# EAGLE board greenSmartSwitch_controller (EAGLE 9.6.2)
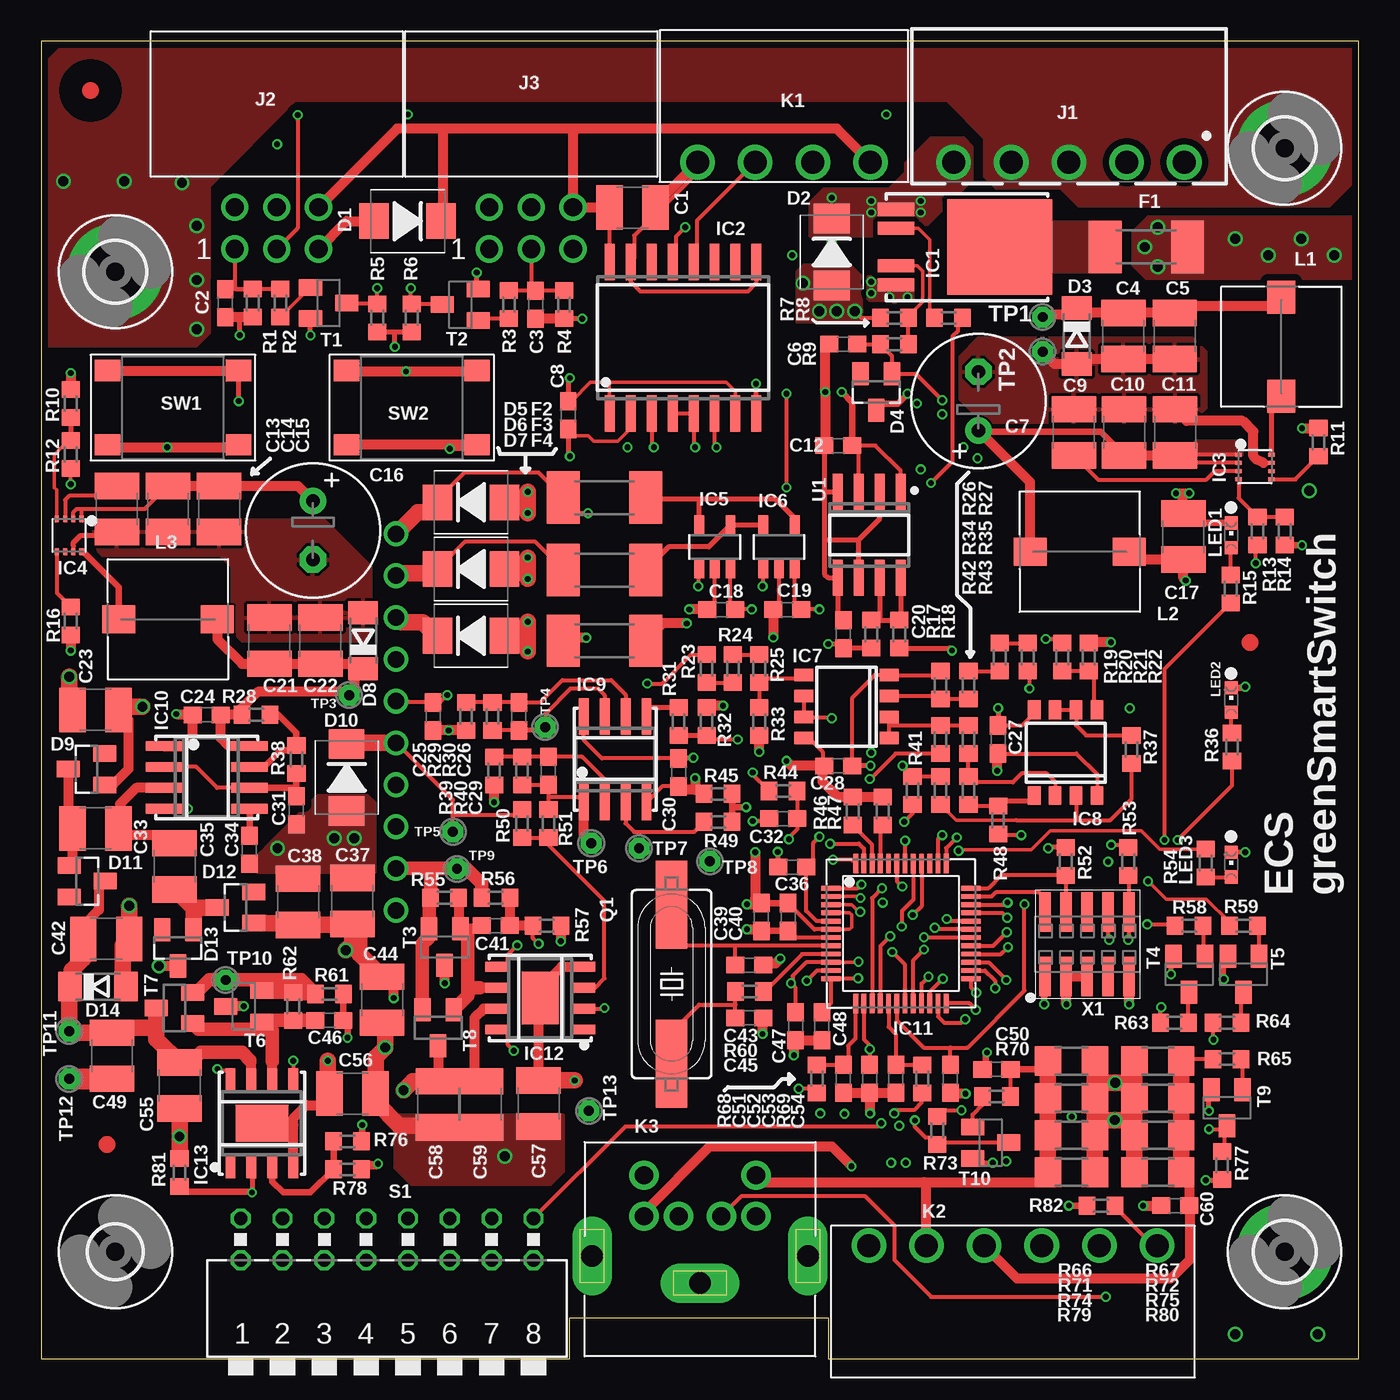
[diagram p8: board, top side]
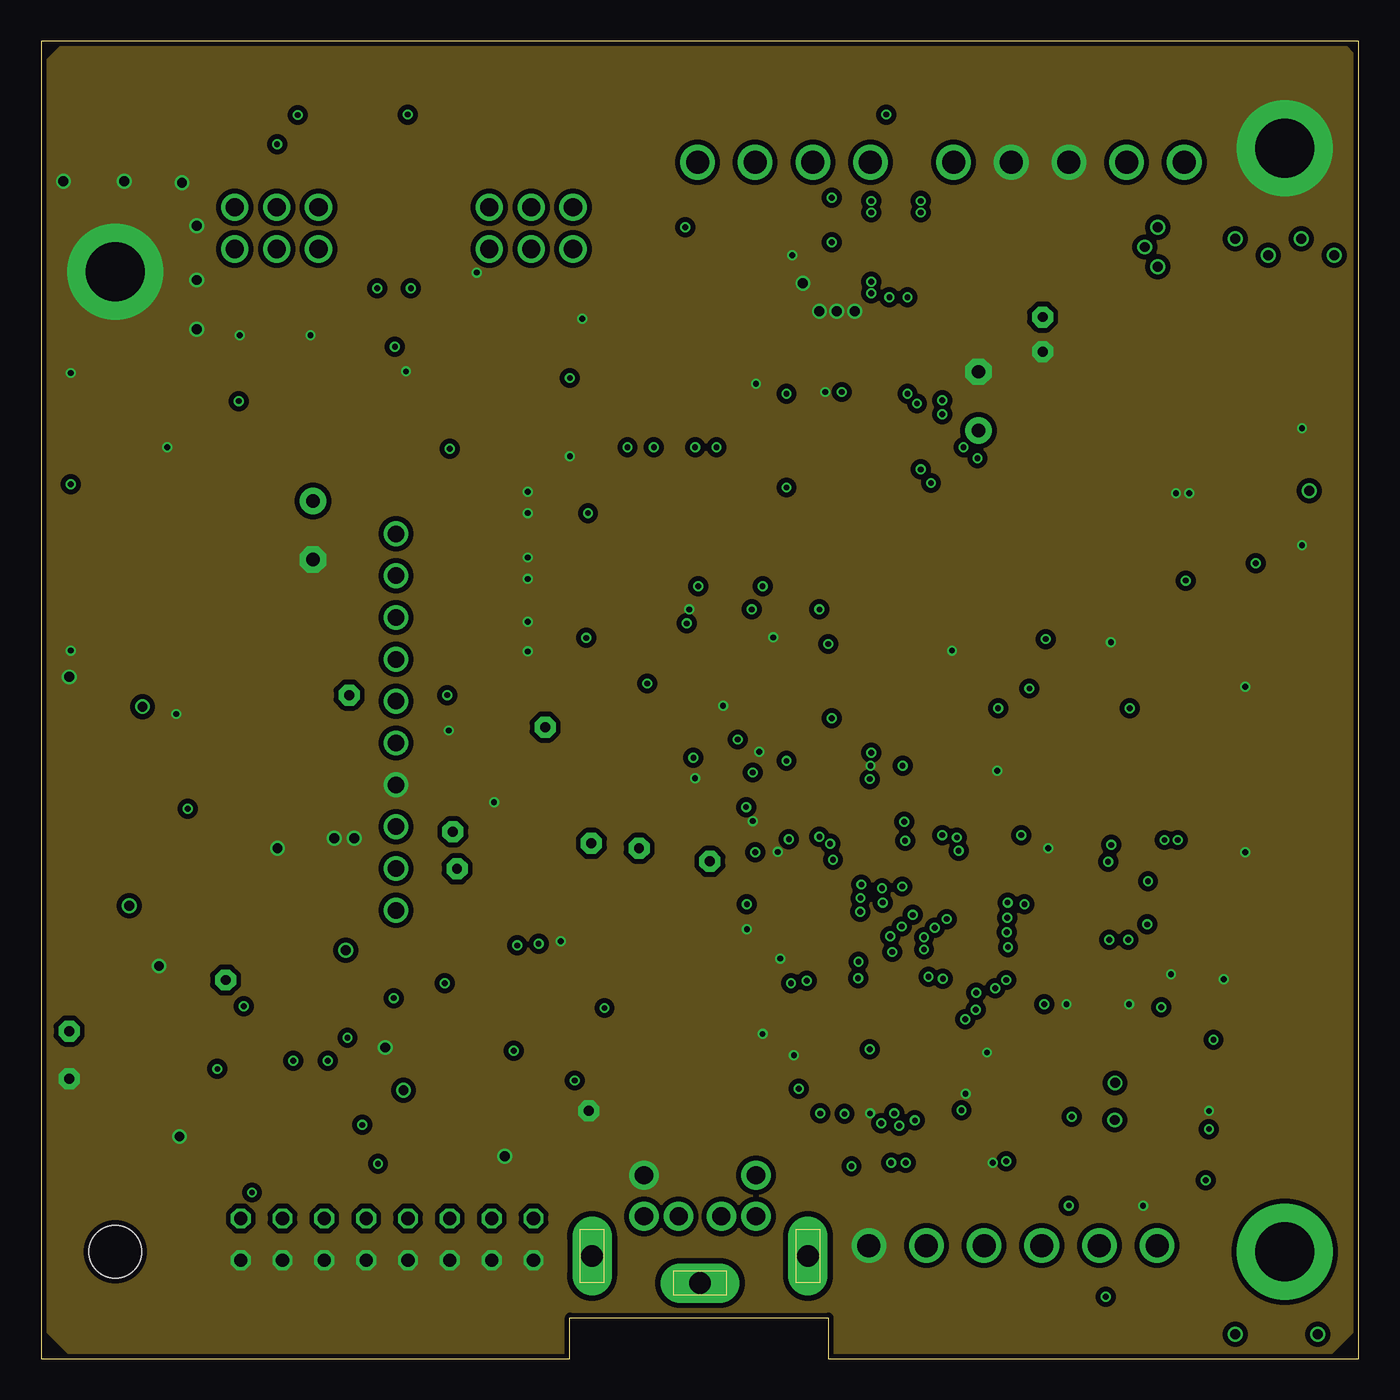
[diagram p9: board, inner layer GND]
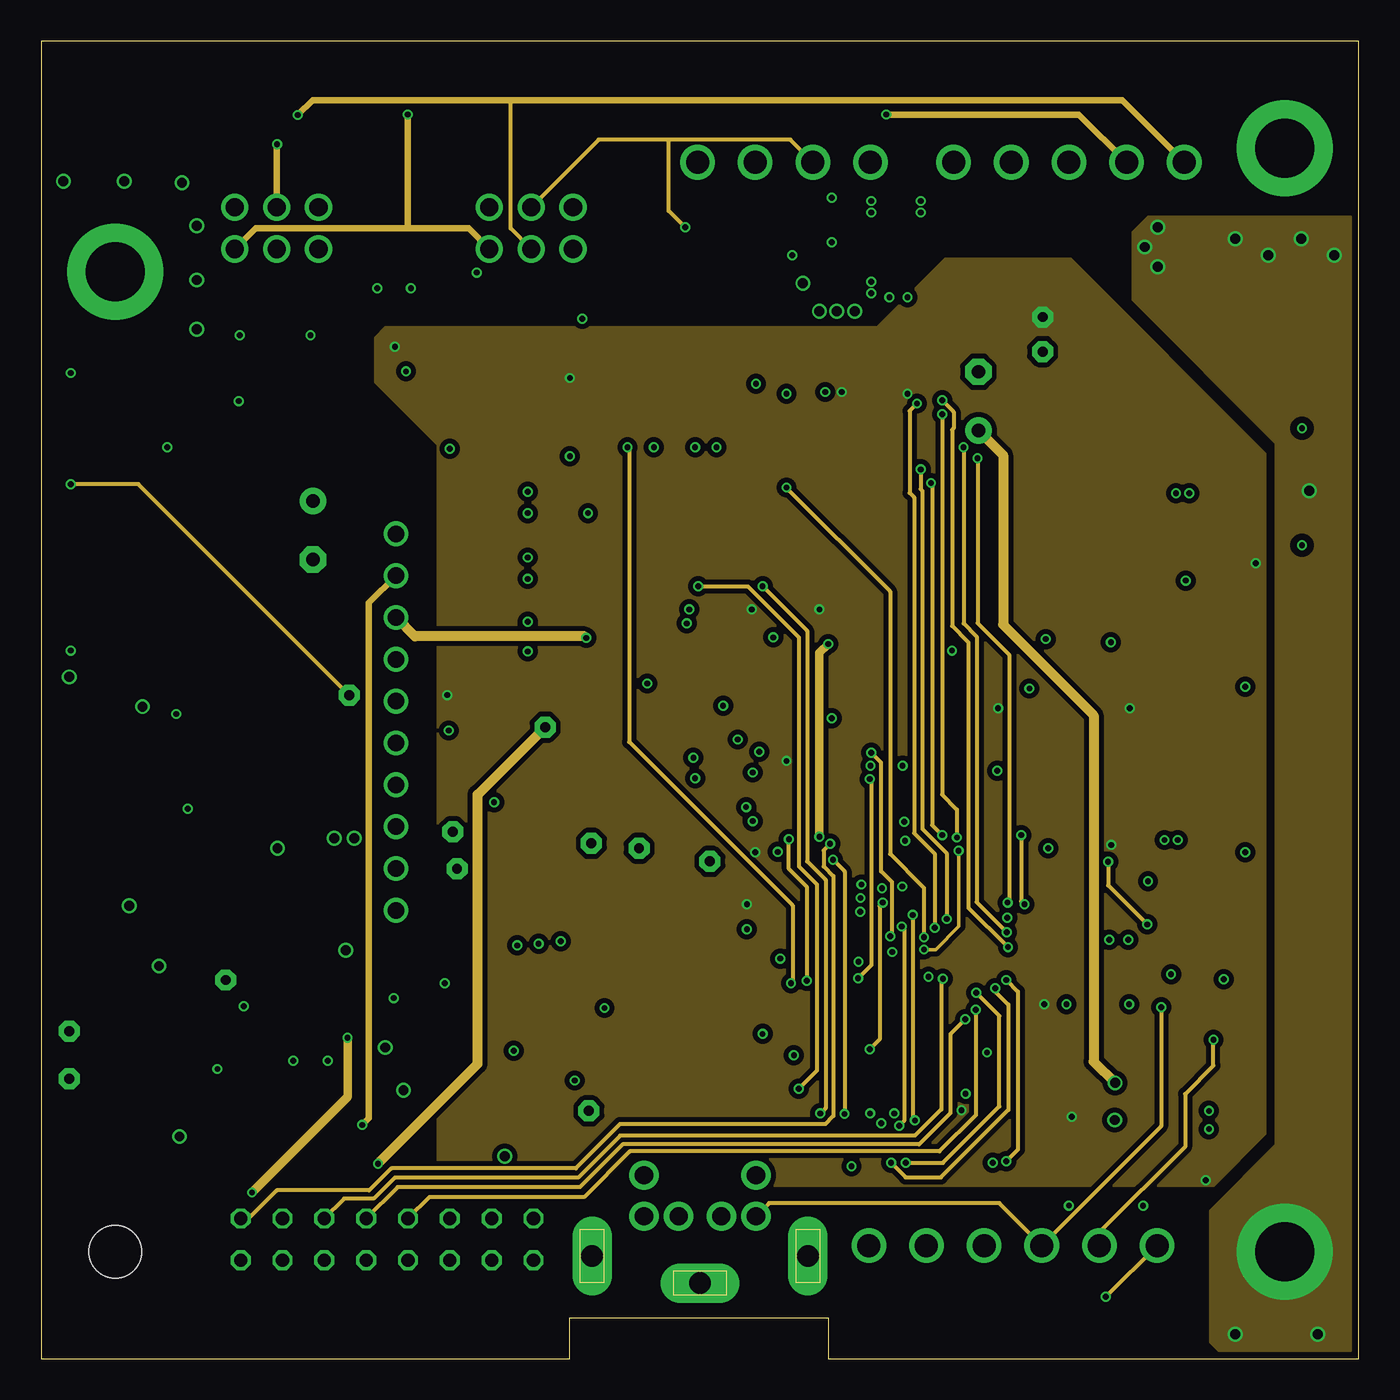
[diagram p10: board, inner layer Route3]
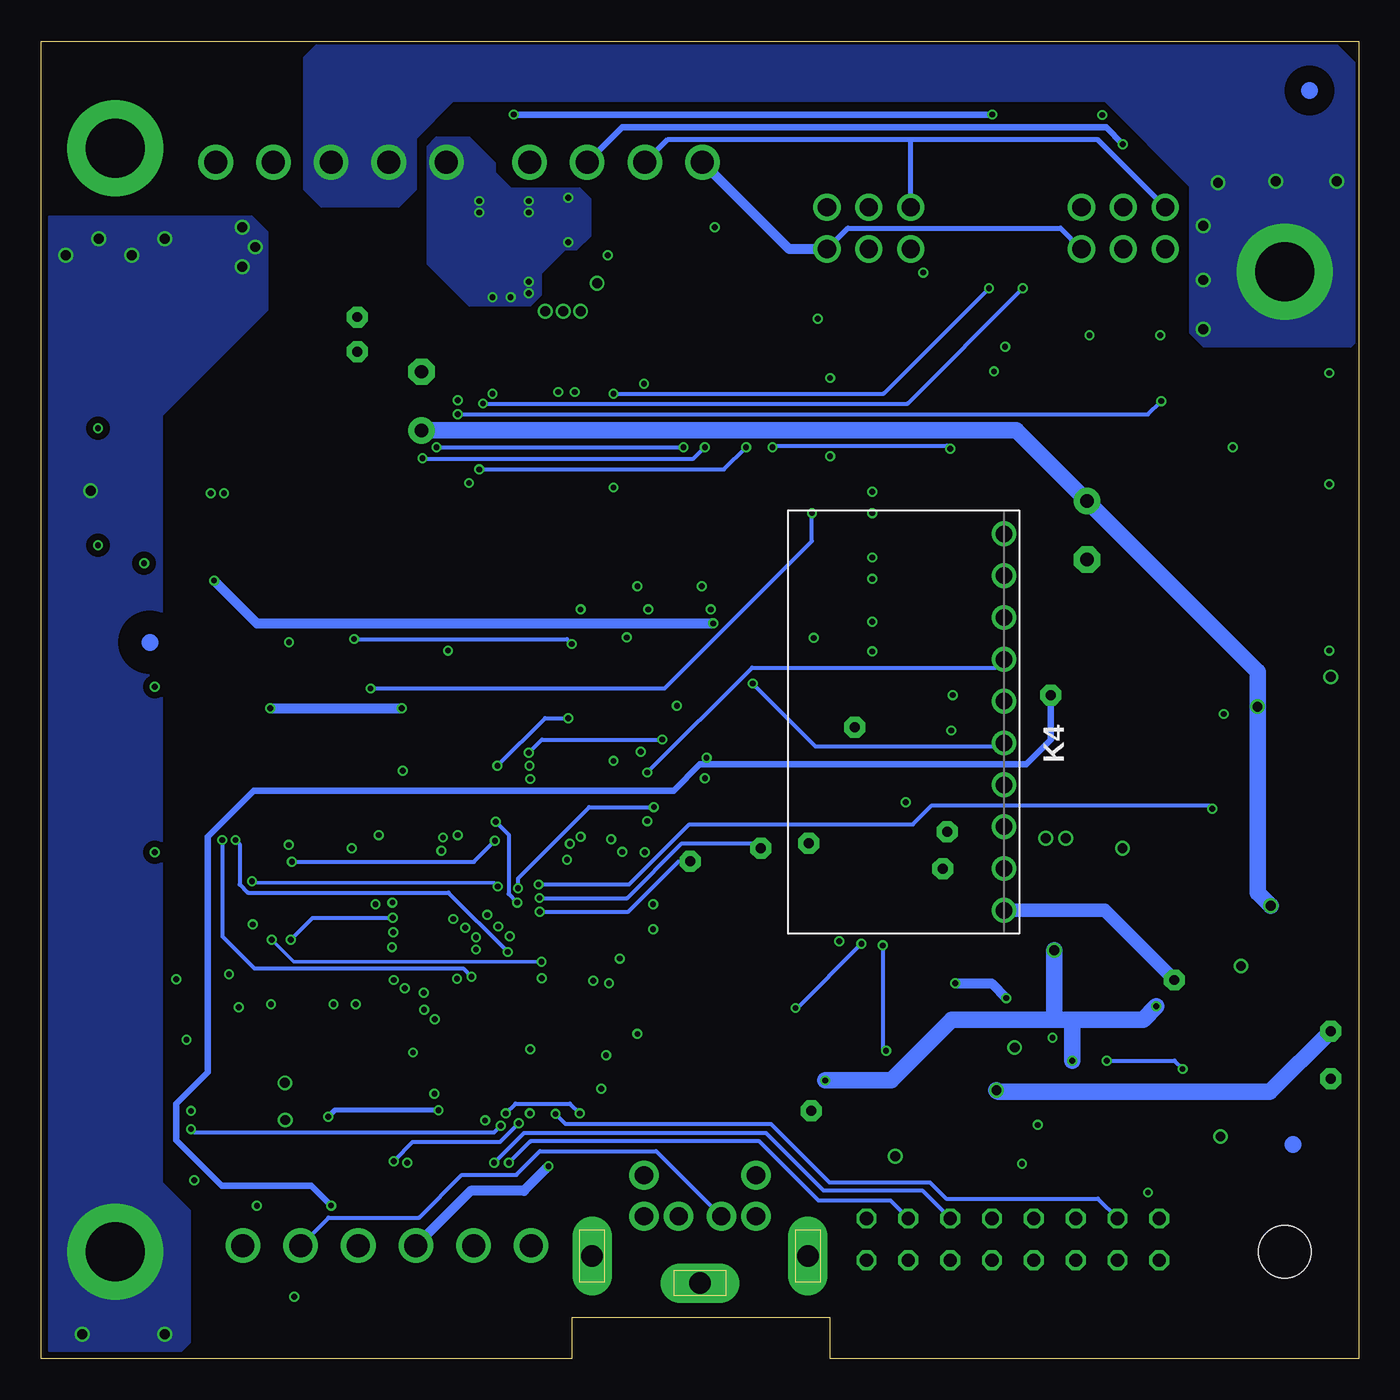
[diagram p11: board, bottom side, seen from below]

Size 80 x 80 mm. Coordinates in mm from the lower left corner, seen from the top.
Outline: 0,0 32.1,0 32.1,2.5 47.8,2.5 47.8,0 80,0 80,80 0,80 0,0
Copper layers (1+2*3+16): Top 0.035mm / dielectric 0.36mm / GND 0.035mm / dielectric 0.7mm / Route3 0.035mm / dielectric 0.36mm / Bottom 0.035mm
Design rules "Multi-CB_4L_125um-Tracks_OL35um-IL35um *": minimum track width 0.125mm, minimum drill 0.2mm, track to track 0.125mm, track to pad 0.125mm, pad to pad 0.125mm, via to via 0.125mm, smd to smd 0mil, copper to edge 0.2mm, drill to drill 0.2mm, minimum pad ring 0.125mm, minimum via ring 0.125mm, stop-mask expansion 2mil, vias tented up to drill 0.45mm, thermal gap 0.2mm

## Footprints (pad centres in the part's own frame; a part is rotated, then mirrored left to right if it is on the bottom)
C1210 = smd 1.6 x 2.7: 1 -1.4,0; 2 1.4,0
C0603 = smd 1.1 x 1: 1 -0.85,0; 2 0.85,0
E3,5-8 = drill 0.813 pad 1.6: + -1.778,0 | drill 0.813 pad 1.6 octagon: - 1.778,0
SMBJ = smd 1.78 x 2.16: A 2.04,0; C -2.03,0
SOD80C = smd 1.4 x 1.8: A 1.7,0; C -1.7,0
SOT23 = smd 1 x 1.4: 1 -0.95,-1.1; 2 0.95,-1.1; 3 0,1.1
SSQ(2410) = smd 2 x 3.18: 1 -2.5,0; 2 2.5,0
3,6-PAD = drill 3.6 pad 5.842: B3,6 0,0
3,2 = hole 3.2: 0,0
PG-TO252-5-11 = smd 0.8 x 2.2: 1 -2.28,-4.2; 2 -1.14,-4.2; 4 1.14,-4.2; 5 2.28,-4.2 | smd 5.8 x 6.4: 3 0,2.1
SO-16DW = smd 0.6 x 2.2: 1 -4.445,-4.6; 2 -3.175,-4.6; 3 -1.905,-4.6; 4 -0.635,-4.6; 5 0.635,-4.6; 6 1.905,-4.6; 7 3.175,-4.6; 8 4.445,-4.6; 9 4.445,4.6; 10 3.175,4.6; 11 1.905,4.6; 12 0.635,4.6; 13 -0.635,4.6; 14 -1.905,4.6; 15 -3.175,4.6; 16 -4.445,4.6
8TDFN = smd 0.25 x 0.4: 1 -0.75,-1; 2 -0.25,-1; 3 0.25,-1; 4 0.75,-1; 5 0.75,1; 6 0.25,1; 7 -0.25,1; 8 -0.75,1
SOT23-5 = smd 0.6 x 1.2: 1 -0.95,-1.306; 2 0,-1.306; 3 0.95,-1.306; 4 0.95,1.306; 5 -0.95,1.306
S8 = smd 0.762 x 1.143: 1 -1.905,-2.6; 2 -0.635,-2.6; 3 0.635,-2.6; 4 1.905,-2.6; 5 1.905,2.6; 6 0.635,2.6; 7 -0.635,2.6; 8 -1.905,2.6
SO8 = smd 0.6 x 2.2: 1 -1.905,-2.6; 2 -0.635,-2.6; 3 0.635,-2.6; 4 1.905,-2.6; 5 1.905,2.6; 6 0.635,2.6; 7 -0.635,2.6; 8 -1.905,2.6
LQFP48 = smd 0.29 x 1.2: 1 -2.75,-4.25; 2 -2.25,-4.25; 3 -1.75,-4.25; 4 -1.25,-4.25; 5 -0.75,-4.25; 6 -0.25,-4.25; 7 0.25,-4.25; 8 0.75,-4.25; 9 1.25,-4.25; 10 1.75,-4.25; 11 2.25,-4.25; 12 2.75,-4.25; 25 2.75,4.25; 26 2.25,4.25; 27 1.75,4.25; 28 1.25,4.25; 29 0.75,4.25; 30 0.25,4.25; 31 -0.25,4.25; 32 -0.75,4.25; 33 -1.25,4.25; 34 -1.75,4.25; 35 -2.25,4.25; 36 -2.75,4.25 | smd 1.2 x 0.29: 13 4.25,-2.75; 14 4.25,-2.25; 15 4.25,-1.75; 16 4.25,-1.25; 17 4.25,-0.75; 18 4.25,-0.25; 19 4.25,0.25; 20 4.25,0.75; 21 4.25,1.25; 22 4.25,1.75; 23 4.25,2.25; 24 4.25,2.75; 37 -4.25,2.75; 38 -4.25,2.25; 39 -4.25,1.75; 40 -4.25,1.25; 41 -4.25,0.75; 42 -4.25,0.25; 43 -4.25,-0.25; 44 -4.25,-0.75; 45 -4.25,-1.25; 46 -4.25,-1.75; 47 -4.25,-2.25; 48 -4.25,-2.75
S8E(SOIC) = smd 0.6 x 1.5: 1 -1.905,-2.6; 2 -0.635,-2.6; 3 0.635,-2.6; 4 1.905,-2.6; 5 1.905,2.6; 6 0.635,2.6; 7 -0.635,2.6; 8 -1.905,2.6 | smd 3.2 x 2.25: 9 0,0
691322110005 = drill 1.4: 1 -7,0; 2 -3.5,0; 3 0,0; 4 3.5,0; 5 7,0
61200621721 = drill 1.1: 1 2.54,1.27; 2 2.54,-1.27; 3 0,1.27; 4 0,-1.27; 5 -2.54,1.27; 6 -2.54,-1.27
691322110004 = drill 1.4: 1 -5.25,0; 2 -1.75,0; 3 1.75,0; 4 5.25,0
691322110006 = drill 1.4: 1 -8.75,0; 2 -5.25,0; 3 -1.75,0; 4 1.75,0; 5 5.25,0; 6 8.75,0
PS/2-6 = drill 1.1 pad 1.778: 1 -1.3,-2; 2 1.3,-2; 3 -3.4,-2; 5 3.4,-2; 6 -3.4,-4.5; 8 3.4,-4.5 | drill 1.3 pad 2.413 long: A1 6.555,0.4; A2 -6.545,0.4; A3 0,2.055
61901011021 = drill 1: 1 1.27,0; 2 -1.27,0; 3 -3.81,0; 4 -6.35,0; 5 -8.89,0; 6 -11.43,0; 7 -13.97,0; 8 -16.51,0; 9 -19.05,0; 10 -21.59,0
WE-PD_7332/7345_PLASTIC_BASE = smd 2 x 1.7: 1 -3,0; 2 3,0
CHIPLED_0603 = smd 0.8 x 0.8: A 0,-0.75; C 0,0.75
HC49UP = smd 5.334 x 1.93: 1 -4.826,0; 2 4.826,0
R0603 = smd 1 x 1.1: 1 -0.85,0; 2 0.85,0
R1206 = smd 1.6 x 1.803: 1 -1.422,0; 2 1.422,0
DA-08 = drill 0.8 octagon: 1 -8.89,-1.27; 2 -6.35,-1.27; 3 -3.81,-1.27; 4 -1.27,-1.27; 5 1.27,-1.27; 6 3.81,-1.27; 7 6.35,-1.27; 8 8.89,-1.27; 9 8.89,1.27; 10 6.35,1.27; 11 3.81,1.27; 12 1.27,1.27; 13 -1.27,1.27; 14 -3.81,1.27; 15 -6.35,1.27; 16 -8.89,1.27
430182095816 = smd 1.55 x 1.3: 1 -3.975,2.25; 2 -3.975,-2.25; 3 3.975,2.25; 4 3.975,-2.25
SOT23-BEC = smd 1 x 1.4: B -0.95,-1.1; C 0,1.1; E 0.95,-1.1
TP_0.6 = drill 0.6 pad 1.27 octagon: TP 0,0
SOIC127P600X175-8N = smd 2.2 x 0.6: 1 -2.6,1.905; 2 -2.6,0.635; 3 -2.6,-0.635; 4 -2.6,-1.905; 5 2.6,-1.905; 6 2.6,-0.635; 7 2.6,0.635; 8 2.6,1.905
PF2X5SMD50MIL = smd 0.7 x 2.4: 1 -2.54,-1.95; 2 -2.54,1.95; 3 -1.27,-1.95; 4 -1.27,1.95; 5 0,-1.95; 6 0,1.95; 7 1.27,-1.95; 8 1.27,1.95; 9 2.54,-1.95; 10 2.54,1.95

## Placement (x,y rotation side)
C1  10µ/16V/X7R  [C1210]  35.9,69.9 180 top
C2  100n  [C0603]  11.18,64.1 90 top
C3  100n  [C0603]  30.02,64 90 top
C4  10µ/16V/X7R  [C1210]  65.7,62.1 90 top
C5  10µ/16V/X7R  [C1210]  68.83,62.1 90 top
C6  100n  [C0603]  48.7,61.6 0 top
C7  220µ/35V  [E3,5-8]  56.9,58.15 90 top
C8  100n  [C0603]  32,57.3 270 top
C9  1µ/100V/X7R  [C1210]  62.7,56.25 270 top
C10  1µ/100V/X7R  [C1210]  65.75,56.25 270 top
C11  1µ/100V/X7R  [C1210]  68.85,56.25 270 top
C12  100n  [C0603]  48.4,55.45 180 top
C13  1µ/100V/X7R  [C1210]  4.6,51.6 90 top
C14  1µ/100V/X7R  [C1210]  7.7,51.6 90 top
C15  1µ/100V/X7R  [C1210]  10.8,51.6 90 top
C16  220µ/35V  [E3,5-8]  16.5,50.3 270 top
C17  1µ/100V/X7R  [C1210]  69.35,49.92 270 top
C18  100n  [C0603]  41.3,45.5 180 top
C19  100n  [C0603]  45.3,45.5 180 top
C20  2µ2/10V/X5R  [C0603]  48.7,44 90 top
C21  10µ/16V/X7R  [C1210]  13.85,43.6 270 top
C22  10µ/16V/X7R  [C1210]  16.95,43.6 270 top
C23  1µ/100V/X7R  [C1210]  3.3,39.4 0 top
C24  100n  [C0603]  10.05,39.1 180 top
C25  100n  [C0603]  23.8,39 270 top
C26  10p  [C0603]  29,39 90 top
C27  100n  [C0603]  58.1,37.6 90 top
C28  100n  [C0603]  48.4,36 180 top
C29  10p  [C0603]  30.8,35.7 90 top
C30  100n  [C0603]  38.7,35.6 270 top
C31  1n  [C0603]  15.5,33.3 90 top
C32  100n  [C0603]  45.05,32.8 180 top
C33  1µ/100V/X7R  [C1210]  3.3,32.2 180 top
C34  10n  [C0603]  12.65,30.9 90 top
C35  1µ/100V/X7R  [C1210]  8.1,29.9 90 top
C36  2µ2/10V/X5R  [C0603]  45.6,29.85 180 top
C37  1µ/100V/X7R  [C1210]  18.9,27.8 90 top
C38  1µ/100V/X7R  [C1210]  15.6,27.75 90 top
C39  2µ2/10V/X5R  [C0603]  43.73,26.82 270 top
C40  2µ2/10V/X5R  [C0603]  45.35,26.82 270 top
C41  47p  [C0603]  27.6,26.3 0 top
C42  1µ/100V/X7R  [C1210]  3.95,25.5 180 top
C43  15p  [C0603]  43,23.9 180 top
C44  1µ/100V/X7R  [C1210]  20.7,21.8 270 top
C45  15p  [C0603]  43,20.7 180 top
C46  47p  [C0603]  17.5,20.55 0 top
C47  100n  [C0603]  45.8,20.2 270 top
C48  100n  [C0603]  47.4,20.2 90 top
C49  1µ/100V/X7R  [C1210]  4.3,18.4 270 top
C50  100n  [C0603]  58,17.57 180 top
C51  10n  [C0603]  48.7,17 90 top
C52  100n  [C0603]  50.3,17 90 top
C53  10n  [C0603]  51.9,17 90 top
C54  10n  [C0603]  55.2,17 90 top
C55  1µ/100V/X7R  [C1210]  8.4,16.6 270 top
C56  1µ/100V/X7R  [C1210]  18.9,16.1 0 top
C57  1µ/100V/X7R  [C1210]  30.2,15.5 270 top
C58  1µ/100V/X7R  [C1210]  24.1,15.45 270 top
C59  1µ/100V/X7R  [C1210]  26.7,15.45 270 top
C60  100n  [C0603]  68.85,9.3 180 top
D1  SMBJ5A  [SMBJ]  22.25,69.07 180 top
D2  SMB15F30A  [SMBJ]  48,67.2 270 top
D3  3V3  [SOD80C]  62.88,62.1 270 top
D4  BAS116  [SOT23]  50.7,58.7 180 top
D5  SMB15F30A  [SMBJ]  26.1,52 0 top
D6  SMB15F30A  [SMBJ]  26.1,47.95 0 top
D7  SMB15F30A  [SMBJ]  26.1,43.9 0 top
D8  13V  [SOD80C]  19.55,43.6 90 top
D9  BAS116  [SOT23]  2.75,35.8 90 top
D10  SMB15F30A  [SMBJ]  18.55,35.3 270 top
D11  BAS116  [SOT23]  2.8,29 270 top
D12  BAS116  [SOT23]  11.8,27.4 90 top
D13  BAS116  [SOT23]  8.3,24.95 180 top
D14  13V  [SOD80C]  3.45,22.6 0 top
F1  10A  [SSQ(2410)]  67.1,67.5 0 top
F2  250mA  [SSQ(2410)]  34.2,52.3 180 top
F3  250mA  [SSQ(2410)]  34.2,47.9 180 top
F4  1A  [SSQ(2410)]  34.2,43.6 0 top
H1  MOUNT-PAD-ROUND3.6  [3,6-PAD]  75.5,73.5 0 top
H2  MOUNT-PAD-ROUND3.6  [3,6-PAD]  4.5,66 0 top
H3  MOUNT-HOLE3.2  [3,2]  4.5,6.5 0 top
H4  MOUNT-PAD-ROUND3.6  [3,6-PAD]  75.5,6.5 0 top
IC1  BTS443  [PG-TO252-5-11]  56.1,67.5 270 top
IC2  ADM2483  [SO-16DW]  38.98,62 0 top
IC3  MAX15062C  [8TDFN]  73.7,54.15 270 top
IC4  MAX15062C  [8TDFN]  1.7,50 180 top
IC5  INA281B  [SOT23-5]  40.9,49.3 0 top
IC6  INA281B  [SOT23-5]  44.8,49.3 0 top
IC7  TSV992  [S8]  48.9,39.6 90 top
IC8  TSV992  [S8]  62.2,36.8 0 top
IC9  TSB712  [SO8]  34.85,36.4 0 top
IC10  TLC555  [SO8]  10.05,35.3 270 top
IC11  STM32G071CBT6TR  [LQFP48]  52.2,25.82 270 top
IC12  LTC6090  [S8E(SOIC)]  30.3,21.9 90 top
IC13  LTC6090  [S8E(SOIC)]  13.4,14.3 0 top
J1  691322110005  [691322110005]  62.4,72.65 180 top
J2  WS6W  [61200621721]  14.3,68.65 180 top
J3  WS6W  [61200621721]  29.75,68.65 180 top
K1  691322110004  [691322110004]  45.1,72.65 0 top
K2  691322110006  [691322110006]  59,6.88 180 top
K3  EB-DIOSM06  [PS/2-6]  40,6.65 180 top
K4  61901011021  [61901011021]  21.55,28.5 270 bottom
L1  47µH/0,85A  [WE-PD_7332/7345_PLASTIC_BASE]  75.3,61.45 90 top
L2  47µH/0,85A  [WE-PD_7332/7345_PLASTIC_BASE]  63.05,49 180 top
L3  47µH/0,85A  [WE-PD_7332/7345_PLASTIC_BASE]  7.7,44.9 0 top
LED1  bl  [CHIPLED_0603]  72.25,50 0 top
LED2  gn  [CHIPLED_0603]  72.25,40 0 top
LED3  rt  [CHIPLED_0603]  72.25,30 0 top
Q1  Q8.000MHz/HC-49SM(SMD)/20pF  [HC49UP]  38.27,22.75 90 top
R1  100k  [R0603]  12.85,64.1 90 top
R2  100k  [R0603]  14.53,64.1 270 top
R3  100k  [R0603]  28.4,64 270 top
R4  100k  [R0603]  31.75,64 90 top
R5  100k  [R0603]  20.4,63.2 270 top
R6  100k  [R0603]  22.5,63.2 270 top
R7  2k2  [R0603]  51.8,63.2 180 top
R8  100R  [R0603]  55.1,63.2 0 top
R9  100R  [R0603]  51.8,61.6 180 top
R10  10k  [R0603]  1.8,58 90 top
R11  0R0  [R0603]  77.55,55.65 90 top
R12  120k  [R0603]  1.8,54.9 90 top
R13  220k  [R0603]  73.85,50.25 90 top
R14  82k  [R0603]  75.5,50.25 270 top
R15  2k2  [R0603]  72.22,46.75 90 top
R16  0R0  [R0603]  1.8,44.8 270 top
R17  22R  [R0603]  50.4,44 90 top
R18  10k  [R0603]  52.1,44 270 top
R19  30k/0,1%  [R0603]  58.2,42.6 90 top
R20  30k/0,1%  [R0603]  59.9,42.6 270 top
R21  10k/0,1%  [R0603]  62,42.6 270 top
R22  10k/0,1%  [R0603]  63.6,42.6 90 top
R23  30k/0,1%  [R0603]  40.4,41.9 90 top
R24  30k/0,1%  [R0603]  42,41.9 270 top
R25  30k/0,1%  [R0603]  43.6,41.9 90 top
R26  10k/0,1%  [R0603]  54.6,40.9 90 top
R27  30k/0,1%  [R0603]  56.3,40.9 90 top
R28  10k  [R0603]  13.05,39.1 0 top
R29  100k  [R0603]  25.8,39 90 top
R30  240k  [R0603]  27.4,39 270 top
R31  100k  [R0603]  38.7,38.7 270 top
R32  100k  [R0603]  40.4,38.7 90 top
R33  10k/0,1%  [R0603]  43.6,38.7 270 top
R34  100R  [R0603]  54.6,37.6 270 top
R35  1k/0,1%  [R0603]  56.3,37.6 270 top
R36  2k2  [R0603]  72.3,37.15 90 top
R37  100k/0,1%  [R0603]  66.2,37 270 top
R38  10k  [R0603]  15.5,36.4 270 top
R39  100k  [R0603]  27.5,35.7 90 top
R40  240k  [R0603]  29.2,35.7 270 top
R41  100R  [R0603]  52.9,34.5 270 top
R42  1k/0,1%  [R0603]  54.6,34.5 270 top
R43  100k/0,1%  [R0603]  56.3,34.5 270 top
R44  100R  [R0603]  45.05,34.48 180 top
R45  100k  [R0603]  41.1,34.3 180 top
R46  3k3  [R0603]  49.27,33.25 90 top
R47  3k3  [R0603]  51.1,33.25 90 top
R48  10R  [R0603]  58.1,32.7 270 top
R49  100k  [R0603]  41.1,32.6 0 top
R50  100k  [R0603]  29.2,32.5 270 top
R51  100k  [R0603]  30.8,32.5 270 top
R52  3k3  [R0603]  62.2,30.2 90 top
R53  10k  [R0603]  66,30.2 90 top
R54  2k2  [R0603]  70.7,30.1 270 top
R55  47R  [R0603]  24.5,28 180 top
R56  100k  [R0603]  27.6,28 0 top
R57  100k  [R0603]  30.7,26.3 0 top
R58  2k2  [R0603]  69.7,26.3 180 top
R59  2k2  [R0603]  73,26.3 180 top
R60  220R  [R0603]  43,22.3 0 top
R61  100k  [R0603]  17.5,22.15 0 top
R62  47R  [R0603]  15.3,21.4 90 top
R63  0R0  [R0603]  68.8,20.4 0 top
R64  0R0  [R0603]  72,20.4 0 top
R65  100k  [R0603]  72,18.2 180 top
R66  4k70  [R1206]  62.55,18.07 0 top
R67  4k70  [R1206]  67.8,18.07 180 top
R68  100R  [R0603]  47.1,17 90 top
R69  100R  [R0603]  53.5,17 90 top
R70  100k  [R0603]  58,15.93 0 top
R71  4k70  [R1206]  62.55,15.82 0 top
R72  4k70  [R1206]  67.8,15.82 180 top
R73  100k  [R0603]  54.4,13.88 90 top
R74  4k70  [R1206]  62.55,13.57 0 top
R75  4k70  [R1206]  67.8,13.57 180 top
R76  100k  [R0603]  18.6,13.2 180 top
R77  100k  [R0603]  71.7,11.75 270 top
R78  100k  [R0603]  18.6,11.5 180 top
R79  4k70  [R1206]  62.55,11.32 0 top
R80  4k70  [R1206]  67.8,11.32 180 top
R81  100k  [R0603]  8.4,11.3 90 top
R82  0R0  [R0603]  64.35,9.3 180 top
S1  418217270908A  [DA-08]  21,7.25 0 top
SW1  [430182095816]  8,57.75 0 top
SW2  [430182095816]  22.5,57.75 180 top
T1  MMBT2222ALT1G  [SOT23-BEC]  17.45,64.1 270 top
T2  MMBT2222ALT1G  [SOT23-BEC]  25.45,64 90 top
T3  FMMT722  [SOT23-BEC]  24.5,25 180 top
T4  MMBT2222ALT1G  [SOT23-BEC]  69.7,23.35 180 top
T5  MMBT2222ALT1G  [SOT23-BEC]  73,23.35 180 top
T6  FMMT722  [SOT23-BEC]  12.3,21.4 90 top
T7  FMMT620  [SOT23]  8.1,21.3 90 top
T8  FMMT620  [SOT23]  24.1,20.1 180 top
T9  MMBT2222ALT1G  [SOT23-BEC]  72,15.25 180 top
T10  MMBT2222ALT1G  [SOT23-BEC]  57.65,13.12 270 top
TP1  TP_0.6  [TP_0.6]  60.8,63.25 270 top
TP2  TP_0.6  [TP_0.6]  60.8,61.15 270 top
TP3  TP_0.6  [TP_0.6]  18.7,40.3 0 top
TP4  TP_0.6  [TP_0.6]  30.6,38.35 0 top
TP5  TP_0.6  [TP_0.6]  25,32 0 top
TP6  TP_0.6  [TP_0.6]  33.4,31.3 180 top
TP7  TP_0.6  [TP_0.6]  36.3,31 0 top
TP8  TP_0.6  [TP_0.6]  40.6,30.2 0 top
TP9  TP_0.6  [TP_0.6]  25.25,29.75 0 top
TP10  TP_0.6  [TP_0.6]  11.2,23 90 top
TP11  TP_0.6  [TP_0.6]  1.7,19.9 0 top
TP12  TP_0.6  [TP_0.6]  1.7,17 0 top
TP13  TP_0.6  [TP_0.6]  33.25,15.05 180 top
U1  MCP1501-30E/SN  [SOIC127P600X175-8N]  50.27,50.02 270 top
U$1  [CIRCLE-1MM-3R]  3,77 0 top
U$2  [CIRCLE-1MM-3R]  73.4,43.5 0 top
U$3  [CIRCLE-1MM-3R]  4,13 0 top
X1  JTAG  [PF2X5SMD50MIL]  63.5,25.18 0 top

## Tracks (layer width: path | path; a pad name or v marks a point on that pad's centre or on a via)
+5V_BUS
  Top 0.254: IC2.16 34.53,69.87 C1.2
  Top 0.61: 32.5,74.69 48.3,74.69 K1.4 | 32.5,74.69 24.4,74.69 | 24.4,74.69 21.61,74.69 J2.6 | D1.C 24.4,69.19 24.4,74.69 | 32.5,74.69 32.29,74.48 J3.6 34.48,69.92 C1.2
+12V  (via drill 0.35)
  Top 0.254: C30.1 34.05,36.45 32.95,37.55 IC9.8 | v1.8,53.1 R12.1
  Top 0.305: v39.6,36.5 39.55,36.45 C30.1
  Top 0.406: v62.4,9.3 R82.2
  Top 0.61: L3.2 10.7,43.7 12.2,42.2 C21.2 C22.2 19.25,42.2 D8.C 19,41.35 19,40.6 TP3.TP 18.5,40.5 13.15,40.5 12.2,39.55 R28.1 C24.1 10.9,37.7 11.39,37.2 IC10.8
  Route3 0.254: TP3.TP 5.9,53.1 v1.8,53.1
  Bottom 0.406: TP3.TP 18.7,37.6 20.2,36.1 39.6,36.1 | 39.6,36.1 40,36.1 41.6,34.5 67.1,34.5 69.9,31.7 69.9,17.4 71.8,15.5 71.8,13.26 69.03,10.49 63.59,10.49 v62.4,9.3 | v39.6,36.5 39.6,36.1
+UB  (via drill 0.6)
  Top 0.254: IC3.1 68.9,54.9 | IC3.2 69.3,54.4 C11.2 | C14.2 6.3,51.6 2.45,51.6 | IC4.2 1.95,51.4 2.15,51.6 2.45,51.6 | IC4.1 2.45,51.6
  Top 0.406: C7.+ 57,56.27 64.33,56.27 C10.2
  Top 0.61: C10.2 C11.2 68.9,54.9 | L2.2 60.05,53.22 C7.+ | C14.2 C15.2 15.58,53 C16.+ | D9.1 4.35,34.85 5.3,35.8 5.3,38.8 C23.2
  Top 1.016: R66.2 63.97,16.7 | 63.97,16.7 R71.2 63.97,14.5 | 63.97,14.5 R74.2 R79.2 | R80.2 R75.2 66.38,14.5 | 63.97,16.7 64.02,16.75 v65.2,16.75 66.33,16.75 66.38,16.8 | 63.97,14.5 v65.17,14.5 66.38,14.5 | R67.2 66.38,16.8 | 66.38,16.8 R72.2 66.38,14.5 | v6.15,39.6 5.3,39.6 5.1,39.4 C23.2 | v5.35,27.5 C42.1 4.95,25.1 4.95,22.8 D14.A
  Route3 0.61: C7.+ 58.4,54.87 58.4,44.57 63.9,39.07 63.9,18.05 v65.2,16.75
  Bottom 1.016: C7.+ 20.79,56.37 C16.+ 6.15,41.73 v6.15,39.6 6.15,28.3 v5.35,27.5
  pour Top (no thermals): 72.9,54.9 72.9,55.6 72.8,55.7 70.1,55.7 70,55.6 70,54.9
A
  Top 0.254: IC2.12 39.81,66.8 39.81,69.11 K1.2
  Bottom 0.305: 27.21,74.05 15.88,74.05 J2.2 | K1.2 41.95,74.05 27.21,74.05 | J3.2 27.21,74.05
B  (via drill 0.35)
  Top 0.254: v39.1,68.7 38.54,68.14 38.54,66.8 IC2.13
  Route3 0.254: K1.3 45.48,74.02 38.1,74.02 | 38.1,74.02 33.85,74.02 J3.4 | v39.1,68.7 38.1,69.7 38.1,74.02
  Route3 0.406: v14.32,73.75 14.3,73.72 J2.4
  Bottom 0.406: K1.3 44.73,74.77 15.35,74.77 v14.32,73.75
BTN1  (via drill 0.35)
  Top 0.254: v55.6,31.65 54.95,31 IC11.37
  Top 0.305: SW1.3 12,59.98 v12,58.15
  Top 0.61: SW1.1 SW1.3
  Route3 0.254: v54.71,57.35 v54.7,57.34 54.7,34.25 55.6,33.35 v55.6,31.65
  Bottom 0.254: v54.71,57.35 12.8,57.35 v12,58.15
DACA  (via drill 0.35)
  Top 0.254: v51.05,28.57 50.45,27.98 IC11.15
  Top 0.406: R45.1 41.95,33.5 | 41.95,33.5 R49.2 | v42.8,33.5 41.95,33.5
  Bottom 0.254: v51.05,28.57 51.05,29.18 46.73,33.5 v42.8,33.5
DACA_
  Top 0.254: IC9.3 35.48,32.52 36,32 39.65,32 R49.1
DACB  (via drill 0.35)
  Top 0.254: v51.55,25.65 50.95,25.05 IC11.16 | v42.3,37.6 40.65,37.6 R32.1
  Top 0.305: R31.2 R32.1
  Route3 0.254: v51.55,25.65 51.65,25.75 51.65,28.95 51,29.6 51,36.2 v50.4,36.8
  Bottom 0.254: v50.4,36.8 49.6,37.6 v42.3,37.6
DACB_
  Top 0.305: IC9.5 36.76,39.55 R31.1
DIP_1  (via drill 0.35)
  Top 0.254: v47.9,31.27 49.65,31.27 49.95,30.98 IC11.47
  Route3 0.254: v47.9,31.27 47.5,30.88 47.5,29.9 48.1,29.3 48.1,14.75 47.6,14.25 35.14,14.25 32.46,11.57 21.26,11.57 19.91,10.22 14.31,10.22 12.61,8.52 S1.16
DIP_2  (via drill 0.35)
  Top 0.254: IC11.48 49.23,30.3 v48.08,30.3
  Route3 0.254: v48.08,30.3 48.77,29.6 v48.77,14.87
  Bottom 0.254: v48.77,14.87 48.17,14.27 35.7,14.27 32.15,10.72 26.05,10.72 25.05,9.72 15.85,9.72 S1.15
DIP_3  (via drill 0.35)
  Top 0.254: v54.75,23.07 53.95,22.27 IC11.22
  Route3 0.254: v54.75,23.07 54.65,22.98 54.65,15.15 53.05,13.55 35.15,13.55 32.6,11 21.47,11 20.19,9.72 18.39,9.72 S1.14
DIP_4  (via drill 0.35)
  Top 0.254: IC11.23 54.45,20.77 54.85,20.38 55.86,20.38 v56.1,20.62
  Route3 0.254: v56.1,20.62 55.2,19.72 55.2,14.92 53.31,13.03 35.3,13.03 32.7,10.43 21.64,10.43 S1.13
DIP_5  (via drill 0.35)
  Top 0.254: IC11.24 56.38,21.57 v56.75,21.2
  Route3 0.254: v56.75,21.2 56.75,14.8 54.54,12.59 35.74,12.59 32.97,9.82 23.57,9.82 S1.12
DIP_6  (via drill 0.35)
  Top 0.254: IC11.25 56.45,22.55 v56.77,22.23
  Route3 0.254: v56.77,22.23 58.17,20.82 58.17,15.32 54.75,11.9 v52.5,11.9
  Bottom 0.254: S1.11 26.51,10.22 32.51,10.22 35.99,13.7 50.7,13.7 v52.5,11.9
DIP_7  (via drill 0.35)
  Top 0.254: IC11.26 57.3,23.57 57.92,22.95 v57.92,22.5
  Route3 0.254: v57.92,22.5 57.92,22.3 58.73,21.5 58.73,15.12 54.62,11.02 52.48,11.02 v51.6,11.9
  Bottom 0.254: S1.10 28.45,9.62 32.82,9.62 36.4,13.2 50.3,13.2 v51.6,11.9
DIP_8  (via drill 0.35)
  Top 0.254: IC11.27 57.52,24.07 v58.6,23 | S1.9 35.47,14.1 50.8,14.1 v51,14.3
  Route3 0.254: v58.6,23 59.3,22.3 59.3,12.7 v58.6,12
  Bottom 0.254: v58.6,12 57.43,13.17 52.13,13.17 v51,14.3
DISABLE_VBOOST  (via drill 0.35)
  Top 0.254: IC11.1 49.58,28.57 v49.8,28.8 | v8.9,33.4 v8.89,33.4 IC10.4
  Bottom 0.254: v8.9,33.4 9.1,33.6 25.92,33.6 27.07,32.45 40.65,32.45 44.3,28.8 v49.8,28.8
GND  (via drill 0.35, 0.6)
  Top 0.2: C8.2 32.4,56.05 33.2,56.05 33.55,55.7 35,55.7 35.8,56.5 IC2.2
  Top 0.254: IC11.7 45.88,25.57 C40.2 | C32.2 44.05,32.65 v43.2,32.65 | IC3.7 74.2,54.4 | C28.1 49.25,40.15 50.6,41.51 IC7.4 54.35,41.51 R26.2 | C19.2 44.8,45.85 IC6.2 | C18.2 40.9,45.95 IC5.2 | C27.1 62.85,36.75 64.11,35.49 IC8.4 | C30.2 37.7,34.75 IC9.4 | 1.95,49.35 IC4.7 | 4.4,50 C13.1 | v49.4,63.6 49.8,63.2 R7.2
  Top 0.305: v44.73,30.77 44.73,29.88 C36.2 | R52.2 61.2,31.05 v61.15,31 | v57.77,11.9 57.75,11.88 56.85,11.88 T10.E | 69.55,56.95 C11.1 | C8.2 32,54.9 v32.1,54.8 | v43.4,59.2 43.4,57.42 IC2.8 | R18.2 55.15,43.15 v55.3,43 | C20.2 48.37,45.18 U1.5 47.77,47.42 47.55,47.65 47.55,49.7 | v50.35,36 C28.1 | T2.E 26.45,65.05 v26.45,65.95 | v16.35,62.15 T1.E | v32.85,63.15 R4.1 | v12.05,62.15 12.05,63.2 12,63.25 | v68.6,23.35 68.6,24.3 T4.E | v71.8,23.05 71.8,24.2 T5.E | v70.9,15.05 70.9,16.2 T9.E | v73.1,30.75 LED3.C | C12.2 47.55,52.6 | U1.4 48.34,52.6 47.55,52.6 | U1.2 50.91,51.01 49.64,49.74 | 47.55,52.6 47.55,49.7 | U1.6 49.64,49.74 | 49.64,49.74 49.6,49.7 47.55,49.7 | 4.4,50 2.4,50 1.95,49.55 1.95,49.35
  Top 0.406: C40.2 C39.2 | C50.2 57.35,17.77 57.35,18.52 v57.42,18.6 | v76.55,49.4 R14.2 | LED2.C 73.05,40.75 v73.1,40.8 | LED1.C 69.92,50.75 C17.1
  Top 0.61: v42.85,26.07 43.62,26.07 C39.2 | X1.5 X1.3 62.25,23.2 v62.25,21.52 | v44.88,24.3 44.58,24 43.95,24 C43.1 | C5.1 C4.1 63.17,60.7 D3.A 61.55,60.4 TP2.TP | v68.9,52.55 69.3,52.55 | 69.3,52.55 v69.7,52.55 | C17.1 69.3,51.37 69.3,52.55 | 74.2,54.4 73.8,54.6 73.6,54.8 73.6,56.3 72.95,56.95 69.55,56.95 | v76.55,56.5 R11.2 | SW2.4 18.68,59.95 v22.15,59.95 26.52,59.95 SW2.2 | SW1.2 4.17,55.35 v7.65,55.35 11.82,55.35 SW1.4 | R1.1 12,63.25 C2.1 | R4.1 C3.1 | v66.9,9.3 C60.2 | v66.05,21.52 66.05,23.21 X1.9 | C48.1 47.25,19.2 47.1,19.35 C47.2 45.7,19.25 v45.7,18.43 | v43.8,19.73 43.8,20.65 C45.1 | v56.12,16.1 55.25,16.1 C54.1 | C51.1 C52.1 | C52.1 C53.1 | v50.33,14.9 50.33,16.12 C52.1 | v64.95,43.5 63.65,43.5 R22.2 | R29.1 v24.75,38.15 C25.2 | C18.2 v39.35,45.5 | C19.2 v44.45,43.8 | v58.05,35.7 58.05,36.7 C27.1 | R45.2 40,34.55 39.7,34.55 | 39.7,34.55 38.9,34.55 C30.2 | v39.7,35.25 39.7,34.55 | R32.2 40.5,39.65 v41.4,39.65 | v27.5,33.8 R39.1 | R57.2 v31.55,25.35 | R16.2 v1.8,43 | v1.8,59.85 R10.2 | IC10.1 8.65,37.2 9.2,37.75 C24.2 9.15,39.15 v8.2,39.15 | v7.15,23.85 D13.3 | v43.6,36.85 R33.2 | C12.2 47.6,55.5 v47.6,58.7 47.6,61.35 C6.1
  Top 1.016: v29.55,51.35 29.55,52 | 29.55,52 v29.55,52.65 | v29.55,47.35 29.55,48 | 29.55,48 v29.55,48.65 | v29.55,42.95 29.55,43.8 | 29.55,43.8 v29.55,44.75 | D6.A 29.5,47.95 29.55,48 | D5.A 29.55,52 | D7.A 29.45,43.9 29.55,43.8 | C44.2 20.9,20.2 v20.9,18.9 20.3,18.3 C56.2 20.3,15.6 21.75,14.15 24,14.15 C58.2 | v1.7,41.4 1.7,39.6 C23.1 | C55.2 v8.4,13.5 R81.2
  Top 1.27: TP12.TP C49.2
  other vias: 5.05,71.5 8.55,71.4 1.35,71.5 9.45,65.5 9.45,62.5 9.45,68.8 48.3,63.6 47.25,63.6 45.6,67 46.25,65.3 19,31.6 28.15,12.3 17.8,31.6 14.35,31
  pour Top: 55.8,58.25 55.8,60.85 56.9,61.95 69.9,61.95 70.7,61.15 70.7,57.75 69.8,56.85 57.2,56.85
  pour GND (isolate 0.305, no thermals): 1.6,80.05 78.8,80.05 80,78.85 80,2.05 78,0.05 2,0.05 0,2.05 0,78.45
  pour Top (isolate 0.305, no thermals): 45.9,66 46.3,66.4 49.1,66.4 49.8,65.7 49.8,62.95 45.9,62.95
  pour Top (isolate 0.406, no thermals): 60,80 79,80 80,79 80,71.8 78.2,70 63,70 61.9,71.1 58,71.1 57.3,71.8 57.3,74.1 55,76.4 15.4,76.4 10.2,71.2 10.2,62.3 9.4,61.5 0.5,61.5 0,62 0,78.4 1.6,80
  pour Bottom (no thermals): 0,62 0,78.4 1.6,80 63,80 64,79 64,71 63,70 58.3,70 57.3,71 57.3,74.1 55,76.4 15.4,76.4 10.2,71.2 10.2,62.3 9.4,61.5 0.5,61.5
  pour Top (no thermals): 21.5,14.8 31.7,14.8 31.7,11.4 30.9,10.6 22.5,10.6 21.5,11.6
  pour Top: 3.5,50.9 17.2,50.9 20,48.1 20,43.9 19.7,43.6 12.2,43.6 11.6,44.2 11.6,48.1 10.9,48.8 3.75,48.8 3.2,49.35 3.2,50.6
  pour Top (isolate 0.406, no thermals): 20.25,29.55 13.15,29.55 13.15,30.55 16.8,34.2 19.8,34.2 20.25,33.75
GND_BUS
  Top 0.254: IC2.9 43.42,65.32 42.9,64.8 36.4,64.8 35.8,65.4 IC2.15 36,66.8 36,68.2 39.85,72.05 K1.1
  Top 0.61: J2.5 18.53,69.07 D1.A | K1.1 37.3,70.1 C1.1
  Bottom 0.305: J3.5 31.02,68.64 18.11,68.64 J2.5
  Bottom 0.61: K1.1 34.58,67.38 J3.5
I_SENSE_CHG
  Top 0.254: IC11.13 49.45,19.45 49,19 49,18.15 C51.2 R68.2
I_SENSE_DISCHG
  Top 0.254: IC11.17 51.45,20.15 51.9,19.7 C53.2 R69.2
LED_ERROR  (via drill 0.35)
  Top 0.2: v55.7,30.85 55.75,30.9 60.1,30.9 61.25,32.05 66.8,32.05 67.9,30.95 R54.1
  Top 0.254: v53.6,24.85 52.95,24.2 IC11.20
  Route3 0.2: v53.6,24.85 54.3,24.85 55.7,26.25 v55.7,30.85
LED_FUNCTION  (via drill 0.35)
  Top 0.254: v51.67,24.7 52.45,23.93 IC11.19 | R15.1 68.2,41.88 v68.2,31.5
  Bottom 0.254: v51.67,24.7 55.27,28.3 67.45,28.3 67.95,28.8 67.95,31.25 v68.2,31.5
LED_STATE  (via drill 0.35)
  Top 0.254: v53.88,23.2 53.45,22.77 IC11.21 | R36.1 72.3,34.8 v69,31.5
  Bottom 0.254: v53.88,23.2 54.38,23.7 67.05,23.7 69,25.65 v69,31.5
LED_SW_ERROR  (via drill 0.35)
  Top 0.254: IC11.42 v52.45,31.45 | v67.15,26.38 68.78,26.38 R58.2
  Route3 0.254: v67.15,26.38 64.78,28.75 v64.78,30.18
  Bottom 0.254: v64.78,30.18 53.73,30.18 v52.45,31.45
LED_SW_STATE  (via drill 0.35)
  Top 0.2: v67.2,29 68.3,27.9 70.75,27.9 72.15,26.5 R59.2
  Top 0.254: v52.27,28.68 51.95,29 IC11.43
  Bottom 0.2: v52.27,28.68 52.5,28.9 67.1,28.9 v67.2,29
LVP_IN  (via drill 0.35)
  Top 0.254: IC11.31 54.35,26.07 v54.25,26.18 | v20.4,65 R5.1 20.35,64.1 T1.C
  Route3 0.254: v53.17,58 52.73,57.55 52.73,52.58 53,52.3 53,31.93 54.25,30.68 v54.25,26.18
  Bottom 0.254: v53.17,58 27.4,58 v20.4,65
LVP_IN_  (via drill 0.35)
  Top 0.254: R2.1 R1.2 | R1.2 11.8,64.95 11.76,64.99 J2.1 | R1.2 C2.2
  Route3 0.406: 22.25,68.64 13.03,68.64 J2.1 | J3.1 25.95,68.64 22.25,68.64 | v22.25,75.55 22.25,68.64 | J1.2 63.01,75.55 v51.3,75.55
  Bottom 0.406: v51.3,75.55 v22.25,75.55
MOSFET_GATE_A
  Top 0.813: T8.2 23.15,25.2 23.55,25.6 T3.E 23.55,27.9 R55.2 23.65,29.72 23.6,29.77 | K4.2 23.6,29.77 | 23.6,29.77 25.23,29.77 TP9.TP 25.85,29.75 26.75,28.85 R56.1
MOSFET_GATE_B
  Top 0.813: T7.2 9.45,22.25 10.2,23 TP10.TP 15.8,23 R61.1 15.4,22.15 R62.2 13.5,22.25 T6.E
  Bottom 0.813: K4.1 15.43,27.23 TP10.TP
N$1  (via drill 0.35)
  Top 0.254: R44.2 43.2,35.48 v43.2,35.6
  Bottom 0.254: v43.2,35.6 36.83,41.97 22.05,41.97 K4.7
N$2
  Top 0.406: R28.2 14.4,39.1 15.5,38 R38.1 15.2,36.95 14.55,36.95 13.54,35.94 IC10.7
N$3
  Top 0.254: R24.1 R25.2
N$4  (via drill 0.35)
  Top 0.254: R65.2 69.35,18.2 R67.1
  Top 0.61: K2.4 59.25,4.88 68.58,4.88 69.72,6.02 69.72,9.28 C60.1 69.7,10.85 R80.1 | K3.5 36.6,8.9 40.6,12.9 48,12.9 v49.2,11.7
  Top 1.016: R67.1 R72.1 R75.1 R80.1
  Bottom 0.61: v49.2,11.7 50.7,10.2 53.92,10.2 K2.4
N$5
  Top 0.254: Q1.2 38.27,25.07 42.2,25.07 | IC11.8 42.2,25.07 | C43.2 42.15,25.02 42.2,25.07
N$6
  Top 0.254: IC3.5 76.15,53.4 R11.1
N$7
  Top 0.254: C45.2 42.15,21.5 | 42.15,21.5 R60.1 | Q1.1 38.27,19.82 39.95,21.5 42.15,21.5
N$8
  Top 0.254: IC3.3 71.25,53.9 70.7,53.35 64.2,53.35 C9.2
N$9  (via drill 0.35)
  Top 0.254: R82.1 65.5,9 65.5,8.9 66.92,7.47 67.15,7.47 K2.1 | K3.1 42.55,9.9 50,9.9 51.8,8.1 51.8,6 54.04,3.76 v64.64,3.76
  Route3 0.254: K2.1 v64.64,3.76
N$10  (via drill 0.35)
  Top 0.254: IC6.1 43.8,47.94 v43.8,46.9 | R69.1 53.45,16.1 53.45,15.55 53,15.1 52,15.1 v51.8,14.9
  Route3 0.254: v43.8,46.9 46.5,44.2 46.5,30.2 47.63,29.07 47.63,15.23 v47.3,14.9
  Bottom 0.254: v51.8,14.9 51.2,15.5 47.9,15.5 v47.3,14.9
N$11
  Top 0.254: IC11.9 46.2,24.57 43.92,22.3 R60.2
N$12
  Top 0.254: R36.2 72.25,38.05 LED2.A
N$13
  Top 0.305: IC6.5 IC5.4 40.54,49.3 38.1,49.3 F3.1
N$14
  Top 0.254: C50.1 R70.2
  Top 0.406: C50.1 60.63,17.57 R66.1
  Top 0.61: 53.6,10.72 43.83,10.72 K3.6 | K2.5 53.75,10.57 53.6,10.72 | 53.6,10.72 60.53,10.72 R79.1
  Top 1.016: R66.1 R71.1 R74.1 R79.1
N$15
  Top 0.254: R64.2 72.85,22.1 T5.C
N$16  (via drill 0.35)
  Top 0.2: IC11.2 49.65,28.07 v49.75,27.98
  Bottom 0.254: v49.75,27.98 44.42,27.98 41.1,31.3 36.6,31.3 TP7.TP
N$17  (via drill 0.35)
  Top 0.254: v71.17,19.38 71.17,20.38 R64.1
  Route3 0.254: K2.2 64.25,7.67 69.45,12.88 69.45,16.07 71.17,17.8 v71.17,19.38
  Bottom 0.254: K3.2 42.66,12.61 49.72,12.61 51.15,11.18 54.45,11.18 57.05,8.57 62.55,8.57 K2.2
N$18  (via drill 0.35)
  Top 0.254: v68,21.35 67.95,21.3 R63.1
  Route3 0.254: v68,21.35 68,14.12 K2.3 58.17,9.45 44.2,9.45 K3.3
N$19  (via drill 0.35)
  Top 0.305: IC13.2 12.8,11.66 v12.8,10.1
  Top 0.406: v12.8,10.1 12.75,10.15 8.75,10.15 8.45,10.45 R81.1 | v18.6,19.5 18.6,20.3 C46.2 R61.2
  Route3 0.508: v18.6,19.5 18.6,15.9 v12.8,10.1
N$20  (via drill 0.6)
  other vias: 67.8,68.7 67,67.5 67.8,66.3 72.5,68 74.5,67 76.5,68 78.5,67 77,52.7 72.5,1.5 77.5,1.5
  pour Bottom (isolate 0.406, no thermals): 66.3,68.4 67.2,69.3 79.5,69.3 80,68.8 80,1 79,0 72,0 71,1 71,9 72.7,10.7 72.7,57.3 66.3,63.7
  pour Top (isolate 0.406, no thermals): 66.3,66.4 66.3,68.4 67.2,69.3 79.5,69.3 80,68.8 80,66.1 79.5,65.6 67.1,65.6
  pour Route3 (isolate 0.406, no thermals): 66.3,68.4 67.2,69.3 79.5,69.3 80,68.8 80,1 79,0 72,0 71,1 71,9 75,13 75,55.6 66.3,64.3
N$21
  Top 0.254: R14.1 R13.2 72.7,52.25 IC3.4
N$22  (via drill 0.35)
  Top 0.254: v34.2,21.3 34.16,21.27 IC12.2 | v30.2,25.2 29.85,25.55 R57.1
  Top 0.61: R57.1 C41.2 R56.2
  Bottom 0.254: v34.2,21.3 34.1,21.3 v30.2,25.2
N$23
  Top 0.61: D9.3 1.65,32.45 C33.2 1.9,30.15 D11.1
N$24
  Top 0.305: 39.95,52.2 36.8,52.2 F2.1 | 39.95,52.2 44.6,52.2 45.75,51.05 IC6.4 | IC5.5 39.95,52.2
N$25
  Top 0.254: R63.2 69.65,22.2 T4.C
N$26
  Top 1.016: D13.1 9.25,27.35 | 9.25,27.35 C35.1 | D12.3 9.3,27.4 9.25,27.35
N$27
  Top 0.254: R58.1 70.55,24.55 T4.B
N$28
  Top 0.254: IC7.1 51.5,38.4 | 51.5,38.4 IC7.2 | R35.1 R34.1 51.55,38.45 51.5,38.4
N$29
  Top 0.254: R40.2 C29.1 30.8,34.1 | 30.8,34.1 R51.1 | IC9.1 32.65,34.1 30.8,34.1
  Top 0.61: TP6.TP 32.95,31.75 IC9.1
N$30
  Top 0.254: T9.B 72.95,18.1 R65.1
N$31
  Top 0.254: R15.2 72.22,49.23 LED1.A
N$32
  Top 0.254: T10.B 56.55,14.82 57.15,15.43 R70.1
N$33
  Top 0.254: T5.B 73.95,26.2 R59.1
N$34
  Top 0.254: R54.2 LED3.A
N$35
  Top 0.203: R2.2 16.32,65.05 T1.B
N$36
  Top 0.406: IC10.5 C34.2
N$37  (via drill 0.35)
  Top 0.254: IC5.1 39.9,47.94 v39.9,46.9 | R68.1 46.85,16.4 v46,16.4
  Route3 0.254: v39.9,46.9 42.9,46.9 46,43.8 46,29.9 47.1,28.8 47.1,17.5 v46,16.4
N$38  (via drill 0.35)
  Top 0.254: IC12.8 28.1,20 28.3,19.8 28.3,19.1 v28.7,18.7 | IC12.5 28.2,23.8 28.3,23.9 28.3,24.5 v28.9,25.1
  Bottom 0.254: v28.9,25.1 28.9,18.9 v28.7,18.7
N$39
  Top 0.61: IC10.3 5.76,34.66 4.8,33.7 4.8,32.3 C33.1 4.7,32.1 5,31.8 7.6,31.8 C35.2
N$40
  Top 0.254: R3.2 26.65,63.15 T2.B
N$41  (via drill 0.35)
  Top 0.254: v52.3,36 52.9,35.4 R41.1 R42.1 | IC7.6 IC7.7 47.94,38.97 v48,38.9
  Bottom 0.254: v52.3,36 49.4,38.9 v48,38.9
N$42  (via drill 0.35)
  Top 0.2: v49.73,27.15 49.62,27.15 49.2,27.57 IC11.3
  Bottom 0.254: v49.73,27.15 44.35,27.15 41.3,30.2 TP8.TP
N$43
  Top 0.254: R29.2 R30.1 C26.2 30.3,39.85 31.65,41.2 34.6,41.2 35.48,40.31 IC9.6
N$44
  Top 0.254: IC8.2 61.56,35.03 61.05,35.55 59.55,35.55 59,35 56.63,35 56.3,35.33 R43.1 R35.2
N$45
  Top 0.2: R42.2 55.55,32.7 59.2,32.7
  Top 0.254: 59.2,32.7 62.8,32.7 | 62.8,32.7 64.9,32.7 66.2,34 R37.2 | IC8.3 62.84,32.73 62.8,32.7
N$46  (via drill 0.35)
  Top 0.254: IC13.8 11.49,17.4 11.39,17.5 10.8,17.5 v10.7,17.6 | v15.3,18.1 IC13.5
  Bottom 0.254: v15.3,18.1 11.2,18.1 v10.7,17.6
N$47  (via drill 0.35)
  Top 0.61: v33.1,43.77 31.7,43.77 F4.1
  Top 1.016: D7.C 23.97,43.9 23.16,44.71 21.85,44.71 K4.8
  Route3 0.61: v33.1,43.77 33,43.87 22.69,43.87 K4.8
N$48
  Top 0.254: IC7.3 54.41,40.23 R26.1 R27.1
N$49
  Top 0.254: R23.1 R24.2
N$50
  Top 0.254: R27.2 R19.1
N$51
  Top 0.254: IC4.8 2.55,49
  Top 0.406: 2.55,49 4.7,46.85 L3.1
N$52
  Top 0.254: R19.2 R20.1
N$54
  Top 0.254: IC12.3 33.63,22.54 34.2,23.1 34.2,27.8 30.8,31.2 R51.2 R50.2
N$55
  Top 0.254: R21.2 R22.1 63.91,41.45 63.91,39.6 IC8.5
N$56  (via drill 0.35)
  Top 0.254: C26.1 R30.2 | TP4.TP 30.6,39.15 32.15,40.7 33.8,40.7 34.22,40.28 IC9.7
  Top 0.305: TP4.TP 30.4,38.15 C26.1
  Top 0.508: v20.45,11.85 20.35,11.75 19.7,11.75 R78.1
  Route3 0.61: TP4.TP 26.5,34.25 26.5,17.9 v20.45,11.85
N$57
  Top 0.254: R33.1 R25.1 43.85,41.3 46.1,41.3 IC7.5
N$58
  Top 0.254: IC4.5 0.95,46.5 R16.1
N$59
  Top 0.406: IC13.3 14.04,10.77 14.7,10.1 16.35,10.1 R78.2 R76.2
N$60
  Top 0.254: C13.2 4,52.4 1.7,52.4 1.45,52.15 IC4.3
N$61
  Top 0.2: IC4.4 0.95,52.75 0.8,52.9 0.8,54.9 1.65,55.75 R12.2
  Top 0.305: R10.1 R12.2
N$66
  Top 0.254: IC9.2 34.22,35.19 32.85,36.55 C29.2 R40.1 R39.2
N$68
  Top 0.2: R7.1 52.65,63.3 53.52,64.17 53.52,66.02 53.18,66.36 IC1.4
  Top 0.254: R9.1 R7.1
N$70
  Top 0.2: R8.1 53.95,63.5 53.95,67.95 53.26,68.64 IC1.2
N$71
  pour Top (no thermals): 64,69 60,69 60,66 64,66
N$91
  Top 0.305: IC3.8 74.7,57.85 L1.1
N$119
  Top 0.305: R17.2 50.91,44.85 | 50.91,44.85 R18.1 52.18,44.93 U1.8 | U1.7 50.91,44.85
N$9999
  Top 0.254: R48.1 56.4,33.55 R43.2
  Top 0.305: R48.1 58.4,33.85 60.3,33.85 IC8.1
NRST  (via drill 0.35)
  Top 0.2: IC11.10 49.6,24.07 v49.62,24.1
  Top 0.254: IC11.10 46.45,24.07 45.62,23.25 45.62,22.9 v45.52,22.8 45.8,22.52 C47.1 | v66,25.45 66.04,25.49 X1.10 66.04,29.31 R53.1
  Top 0.305: SW2.1 26.23,55.25 v24.8,55.25
  Top 0.61: SW2.1 SW2.3
  Route3 0.254: v45.52,22.8 45.62,22.9 45.62,27.52 35.7,37.45 35.7,55.25 v35.6,55.35
  Bottom 0.2: v66,25.45 64.65,24.1 v49.62,24.1
  Bottom 0.254: v35.6,55.35 35.5,55.45 25,55.45 v24.8,55.25
OUT_CS  (via drill 0.35)
  Top 0.254: IC11.28 58.27,24.57 v58.7,25 | C6.2 R9.2 51.65,60.9 D4.1 53.1,59.8 v54.7,58.2
  Route3 0.254: v58.7,25 56.3,27.4 56.3,43.5 55.3,44.5 55.3,56.4 55.4,56.5 55.4,57.5 v54.7,58.2
OUT_CTRL  (via drill 0.35)
  Top 0.254: IC11.38 54.45,31.55 v54.7,31.8 | v54.02,53.17 55.33,54.48 55.33,62.08 55.65,62.4 55.65,62.9 R8.2
  Route3 0.254: v54.02,53.17 54.1,53.1 54.1,32.4 v54.7,31.8
OUT_CTRL+  (via drill 0.35)
  other vias: 50.4,70.3 50.4,69.6 53.4,69.6 53.4,70.3 48,67.8 48,70.5 51.5,64.45 52.6,64.45 50.4,65.4 50.4,64.7
  pour Top (isolate 0.305, no thermals): 46.7,68.2 46.7,70.2 47.5,71 51.5,71 52.5,72 52.5,72.6 54,74.1 56,74.1 56.5,73.6 56.5,71.6 53.1,68.2
  pour Bottom (no thermals): 46.7,68.2 46.7,70.4 47.3,71 51.5,71 52.5,72 52.5,72.6 54,74.1 56,74.1 56.5,73.6 56.5,66.5 54,64 50.3,64 49.7,64.6 49.7,65.9 48.2,67.4 47.5,67.4
  pour Top (isolate 0.406, no thermals): 50.2,65.7 52.9,65.7 53,65.6 53,64.25 52.85,64.1 50.45,64.1 50.2,64.35
OVP_IN  (via drill 0.35)
  Top 0.254: IC11.30 53.62,25.57 v53.6,25.6 | v45.25,58.6 v45.25,52.9 | v22.45,65 22.45,64.1 R6.1 24.3,64.05 T2.C
  Route3 0.254: v53.6,25.6 53.6,28.6 51.55,30.65 51.55,46.6 v45.25,52.9
  Bottom 0.254: v45.25,58.6 28.85,58.6 v22.45,65
OVP_IN_  (via drill 0.35)
  Top 0.254: v15.57,75.52 15.57,68.66 J2.3 | R4.2 C3.2 29.8,64.85 | 29.8,64.85 R3.1 | J3.3 29.75,64.9 29.8,64.85
  Route3 0.254: 28.5,76.42 28.5,68.63 J3.3
  Route3 0.406: J1.1 65.63,76.42 28.5,76.42 16.48,76.42 v15.57,75.52
PREDRIVER_A
  Top 0.61: C41.1 26.55,26.1 T3.B 25.35,26.2 R55.1 | IC12.6 26.64,22.54
  Top 0.813: 26.64,22.54 26.18,22.54 25.89,22.23 | T8.1 25.89,22.04 25.89,22.23 | T3.B 25.89,25.66 25.89,22.23
PREDRIVER_B
  Top 0.61: IC13.6 14.04,18.07
  Top 0.813: T6.B 13.3,20.35 13.6,20.35 | 14.04,18.07 14.04,19.91 13.95,20 | 13.95,20 13.6,20.35 | 13.6,20.35 13.4,20.55 R62.1 C46.1 | T7.1 9.55,20 13.95,20
R2  (via drill 0.35)
  Top 0.254: X1.8 64.77,25.53 v64.85,25.45 | v58.65,26.77 58.35,27.07 IC11.33
  Bottom 0.254: v58.65,26.77 63.52,26.77 v64.85,25.45
REF_1V5
  Top 0.254: IC8.7 IC8.6 62.84,38.47 63.45,37.85 R37.1
RS485_RX  (via drill 0.35)
  Top 0.254: IC11.32 55.1,26.57 v54.98,26.7 | v37.2,55.35 37.07,55.48 IC2.3
  Route3 0.254: v53.4,54 53.4,52.8 53.5,52.7 53.5,32.17 54.98,30.7 v54.98,26.7
  Bottom 0.254: v37.2,55.35 38.55,54 v53.4,54
RS485_TX  (via drill 0.35)
  Top 0.254: v58.62,25.9 57.8,25.07 IC11.29 | IC2.6 40.88,55.47 v41,55.35
  Route3 0.254: v58.62,25.9 56.8,27.73 56.8,43.85 56,44.65 v56,55.35
  Bottom 0.254: v56,55.35 v41,55.35
RS485_TX_EN  (via drill 0.35)
  Top 0.254: v58.67,27.7 58.55,27.57 IC11.34 | v39.7,55.35 39.61,55.44 IC2.5 IC2.4
  Route3 0.254: v56.85,54.67 56.85,44.67 58.77,42.75 58.77,27.8 v58.67,27.7
  Bottom 0.254: v56.85,54.67 56.83,54.65 40.4,54.65 v39.7,55.35
SCL
  Top 0.254: R47.1 50.95,32.25 IC11.45
SDA
  Top 0.254: IC11.46 50.45,31.23 R46.1
SENSE_A  (via drill 0.35)
  Top 0.254: v36.8,41 37.7,41 39.45,42.75 R23.2 | TP5.TP 25,33 | 25,33 25,33.94 K4.5 | R50.1 28.85,33 25,33
  Top 1.016: D10.C 18.61,37.39 K4.5
  Bottom 0.254: K4.5 21.75,37.19 32.99,37.19 v36.8,41
SENSE_B  (via drill 0.35)
  Top 0.254: D5.C 24.07,52.17 25.7,53.8 30.2,53.8 F2.2 | R20.2 60,41.65 v60,40.7
  Top 0.305: F2.2 31.7,51.35 v33.2,51.35
  Top 1.016: K4.10 22.86,51.4 24.07,51.4 D5.C
  Bottom 0.254: v60,40.7 42.15,40.7 33.2,49.65 v33.2,51.35
SENSE_B_MOSFET  (via drill 0.35)
  Top 0.254: F3.2 30,49.6 25.72,49.6 D6.C
  Top 0.406: R76.1 19.5,13.25 v19.5,14.2
  Top 1.016: K4.9 21.7,47.7 24.01,47.7 D6.C
  Route3 0.406: v19.5,14.2 19.9,14.6 19.9,45.9 K4.9
SENSE_TEMP  (via drill 0.35)
  Top 0.254: IC11.11 47.1,23.57 v46.48,22.95 | v45.4,31.55 45.4,31.65 45.9,32.15 C32.1 R44.1
  Route3 0.254: v46.48,22.95 46.48,28.68 45.4,29.75 v45.4,31.55
SW_OFF  (via drill 0.35)
  Top 0.254: T10.C 54.5,13.12 R73.1 54,13.43 53.7,13.43 53.05,14.07 v53.05,14.47 | IC11.40 53.45,27.48 v52.92,26.95
  Route3 0.254: v52.92,26.95 52.92,14.6 v53.05,14.47
SW_ON  (via drill 0.35)
  Top 0.254: IC11.41 52.95,27.88 52.25,27.18 v52.25,26.25 | v70.9,13.95 71.8,13.95 71.88,14.03 | 71.88,14.03 T9.C | R77.1 71.88,12.78 71.88,14.03
  Route3 0.254: v52.25,26.25 52.4,26.1 52.4,14.45 v52.1,14.15
  Bottom 0.254: v52.1,14.15 52.5,13.75 70.7,13.75 v70.9,13.95
SWCLK
  Top 0.254: X1.4 62.2,27.16 R52.1 58.3,29.35 57.52,28.57 IC11.36
SWDIO
  Top 0.254: IC11.35 57.7,28.07 57.95,28.32 60.56,28.32 60.96,27.93 X1.2
TR
  Top 0.254: IC10.6 10.69,34.66 9.41,35.94 IC10.2
  Top 0.406: C31.2 15.5,34.4 | 15.5,34.4 R38.2 | IC10.6 15.23,34.66 15.5,34.4
U_A_SENSE  (via drill 0.35)
  Top 0.254: IC11.14 49.95,19.4 50.3,19.05 v50.3,18.8 C52.2 | R41.2 52.9,33.1 v52.4,32.6
  Route3 0.254: v51.1,27.7 50.9,27.5 50.9,19.4 v50.3,18.8
  Bottom 0.254: v52.4,32.6 51.62,31.82 51.62,28.23 v51.1,27.7
U_AB_SENSE  (via drill 0.35)
  Top 0.254: IC11.18 51.95,20.55 53.6,18.9 55.2,18.9 | v59.5,31.8 58.15,31.8 R48.2 | v59.7,27.6 59.7,22.35 56.25,18.9 55.2,18.9 | C54.2 55.2,18.9
  Route3 0.254: v59.5,31.8 59.5,27.8 v59.7,27.6
U_BAT  (via drill 0.35)
  Top 0.61: L2.1 66.53,48.52 C17.2 69.35,47.4 v69.5,47.25 | v39.2,44.65 37.75,44.65 F4.2
  Bottom 0.61: v69.5,47.25 66.9,44.65 v39.2,44.65
U_BAT_SENSE  (via drill 0.35)
  Top 0.254: v49.6,23.1 49.58,23.07 IC11.12 47.95,21.6 C48.2 | v50.3,35.2 50.33,35.2 51.88,36.75 R34.2
  Route3 0.254: v49.6,23.1 50.4,23.9 50.4,35.1 v50.3,35.2
V-  (via drill 0.35, 0.6)
  Top 0.61: v24.5,22.8 T3.C | v12.3,21.4 T6.C | 17.4,16.2 C56.1 16.8,15.4 16.1,15.4 15.3,14.61 15.3,14.2 | IC13.4 15.3,14.2 | IC13.9 15.21,14.3 15.3,14.2 | C57.1 30.2,21.8 IC12.9 30.3,22.5 31.61,23.8 IC12.4 | v21.4,21.9 21.4,23.2 C44.1
  Top 1.016: v32.4,16.9 C57.1 | v17.4,18.1 17.4,16.2 | D12.1 15.5,26.45 C38.1 18.85,26.35 C37.1 | C37.1 18.9,25.2 v18.5,24.8 | C44.1 19.3,24.6 19.3,25.8 18.9,26.2 C37.1
  Bottom 0.61: v24.5,22.8 22.3,22.8 v21.4,21.9
  Bottom 1.016: 17.4,20.6 13.1,20.6 v12.3,21.4 | 17.4,20.6 18.5,20.6 | 18.5,20.6 24.7,20.6 28.4,16.9 v32.4,16.9 | v17.4,18.1 17.4,20.6 | v18.5,24.8 18.5,20.6
V_BOOST  (via drill 0.6)
  Top 0.61: IC13.7 12.77,18 12.66,18.1 12.66,18.14 | IC12.7 26.86,21.27 26.3,20.7 26.3,17.25 C59.1 | T8.3 C58.1 | D11.3 3.5,28.6 3.5,27.25 2.55,26.3 C42.2
  Top 0.813: C55.1 9.1,18 9.7,18.6 12.2,18.6 12.66,18.14
  Top 1.016: v22,16.3 22.55,16.85 C58.1 C59.1 | C42.2 2.55,24.3 1.85,23.6 1.85,22.7 D14.C 1.7,22.55 TP11.TP 1.8,19.8 C49.1 4.6,20.1 7,20.1 | C55.1 7,19.4 7,20.1 | 7,20.1 T7.3
  Bottom 1.016: v22,16.3 21.9,16.2 5.4,16.2 TP11.TP
VCC  (via drill 0.35)
  Top 0.2: IC11.6 49.08,26.07 49.2,26.2 49.2,26.95 49.08,27.07 IC11.4 | C8.1 32.2,58.15 33.35,59.3 34.5,59.3 | IC2.7 42.15,58.75 41.6,59.3 34.5,59.3 | IC2.1 34.5,57.43 34.5,59.3
  Top 0.254: IC11.6 46.95,26.07 C40.1 | v73.75,48.3 73.75,49.3 R13.1 | IC7.8 46.6,37.7 47.45,36.84 47.45,36.1 47.45,35.9 | IC6.3 45.75,45.9 C19.1 v47.25,45.5 | IC5.3 41.85,45.8 C18.1 v43.15,45.5 | R73.2 54.77,15.1 v55.88,15.1 | U1.3 49.64,55.06 C12.1 50.65,55.45 52.18,53.92 U1.1 | v64.97,31.2 65.78,31.2 65.92,31.05 R53.2 | IC8.8 60.3,39.2 59.55,38.45 C27.2 | K4.6 21.63,39.85 C25.1 24.2,39.85 v24.65,40.3
  Top 0.305: v32.1,59.55 32,59.45 C8.1 | R5.2 21.5,62.35 | 21.5,62.35 R6.2 | v21.48,61.45 21.48,62.33 21.5,62.35 | v70.7,10.85 71.65,10.85 R77.2 | v58.1,39.5 C27.2
  Top 0.406: C40.1 C39.1 | X1.1 60.9,23.16 v60.9,21.52 | D4.3 51.1,58 52,58 v52.6,58.6 | v48.6,58.7 49.25,58.05 C12.1
  Top 0.61: R47.2 R46.2 48.4,34.1 47.45,35.05 47.45,35.9 | v43.35,30.75 43.35,27.95 43.62,27.68 C39.1 43.65,27.6 v42.85,27.6 | TP1.TP 60.95,63.4 62.48,63.4 D3.C 63.17,63.5 C4.2 C5.2 69.22,63.9 74.75,63.9 L1.2 | 47.45,36.1 47.65,36.1 C28.2 45.55,36 v45.25,36.3
  Bottom 0.305: v55.88,15.1 62.17,15.1 v62.58,14.7
  Bottom 0.61: v66.1,39.5 v58.1,39.5
  pour Route3 (isolate 0.305, no thermals): 62.5,66.75 74.3,54.95 74.3,13.65 71.2,10.55 24.1,10.55 24.1,55.5 20.3,59.3 20.3,62 20.9,62.6 29,62.6 50.75,62.6 54.9,66.75
VREF  (via drill 0.35)
  Top 0.254: IC11.5 47.08,26.57 46.45,27.2 C36.1 46.85,30.25 46.85,31.3 v47.25,31.7 | R21.1 61.75,43.7 v61,43.7
  Top 0.305: R17.1 C20.1 48.45,43.4 v47.78,43.4
  Route3 0.508: v47.78,43.4 47.25,42.87 v47.25,31.7
  Bottom 0.254: v61,43.7 48.08,43.7 v47.78,43.4

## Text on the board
tPlace: ECS | greenSmartSwitch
